(* Logix 5000 AddOnInstructionDefinition export SPEL_XYLimGet; software revision 30.01 *)

ADD_ON_INSTRUCTION SPEL_ExecCmd   (* revision 1.2 *)
// Executes a command in the robot controller.  Normally this is called by higher level AOIs.
VAR_INPUT
   Start : BOOL; {required}
   MaxTime : DINT := 3000; {required}
END_VAR
VAR_OUTPUT
   InCycle : BOOL; {access Read Only, visible}
   Done : BOOL; {access Read Only, visible}
   Error : BOOL; {access Read Only, visible}
END_VAR
VAR_IN_OUT
   ExtInputs : AB:ETHERNET_MODULE_INT_128Bytes:I:0; {required}
        .DATA[0].0   // ExtCmdGet
        .DATA[0].1   // ExtRespSet
        .DATA[0].2   // ExtCmdResult
        .DATA[0].3   // ExtError
   ExtOutputs : AB:ETHERNET_MODULE_INT_128Bytes:O:0; {required}
        .DATA[0].0   // ExtCmdSet
        .DATA[0].1   // ExtRespGet
        .DATA[0].2   // ExtCmdReset
END_VAR
VAR_INPUT
   Cmd : INT; {required}
   CmdParam1 : INT; {required}
   CmdParam2 : INT; {required}
   CmdParam3 : INT; {required}
   CmdParam4 : INT; {required}
   CmdParam5 : INT; {required}
   CmdParam6 : INT; {required}
   CmdParam7 : INT; {required}
END_VAR
VAR_OUTPUT
   CmdEcho : INT; {access Read Only, visible}
   Resp1 : INT; {access Read Only, visible}
   Resp2 : INT; {access Read Only, visible}
   Resp3 : INT; {access Read Only, visible}
   Resp4 : INT; {access Read Only, visible}
   Resp5 : INT; {access Read Only, visible}
   Resp6 : INT; {access Read Only, visible}
   Resp7 : INT; {access Read Only, visible}
   ErrCode1 : INT; {access Read Only, visible}
   ErrCode2 : INT; {access Read Only, visible}
END_VAR
VAR
   ExtReset : BOOL; {access None}
   ExtError : BOOL; {access None}
   ExtCmdSet : BOOL; {access None}   // Cmd Ready
   ExtCmdGet : BOOL; {access None}   // Cmd Received
   CmdXferDone : BOOL; {access None}
   ExtRespSet : BOOL; {access None}   // Resp Ready
   RespXferDone : BOOL; {access None}
   ExtCmdResult : BOOL; {access None}   // Normal or Error?
   TmrCmdDataRdy : TIMER := (PRE := 5); {access None}
   OneShotDoneOff : BOOL; {access None}
   OneShotStart : BOOL; {access None}
   StartInit : BOOL; {access None}
   OneShotStartError : BOOL; {access None}
   TmrCycle : TIMER := (PRE := 5000); {access None}
   OneshotTmrPreset : BOOL; {access None}
   TmrCmdSet : TIMER := (PRE := 20); {access None}
   OnShotCmdDataXfer : BOOL; {access None}
   OneShotRespDataXfer : BOOL; {access None}
   OneShotDataRdy : BOOL; {access None}
   OtherCmdInCycle : BOOL; {access None}
   s : BOOL; {access None}
   OneShotUnsetCmdIncycle : BOOL; {access None}
   OneShotSetCmdIncycle : BOOL; {access None}
   OneShotSetOtherCmdInCycleError : BOOL; {access None}
   OneShotSetBit : BOOL; {access None}
   MaxTimeError : BOOL; {access None}
END_VAR

ROUTINE Logic   (* ladder *)
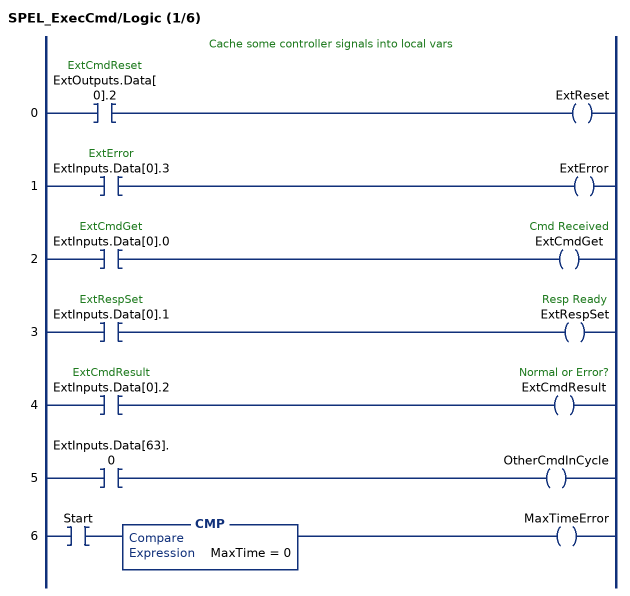
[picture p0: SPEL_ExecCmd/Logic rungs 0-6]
   // Cache some controller signals into local vars
   0: XIC(ExtOutputs.Data[0].2)OTE(ExtReset);
   1: XIC(ExtInputs.Data[0].3)OTE(ExtError);
   2: XIC(ExtInputs.Data[0].0)OTE(ExtCmdGet);
   3: XIC(ExtInputs.Data[0].1)OTE(ExtRespSet);
   4: XIC(ExtInputs.Data[0].2)OTE(ExtCmdResult);
   5: XIC(ExtInputs.Data[63].0)OTE(OtherCmdInCycle);
   6: XIC(Start)CMP(MaxTime = 0)OTE(MaxTimeError);
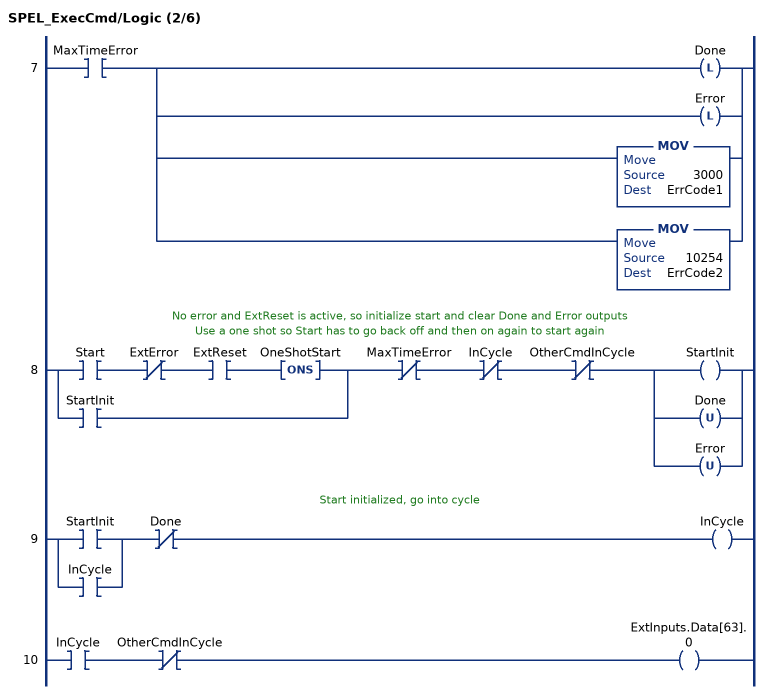
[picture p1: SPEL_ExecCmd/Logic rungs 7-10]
   7: XIC(MaxTimeError)[OTL(Done) ,OTL(Error) ,MOV(3000,ErrCode1) ,MOV(10254,ErrCode2) ];
   // No error and ExtReset is active, so initialize start and clear Done and Error outputs
   // Use a one shot so Start has to go back off and then on again to start again
   8: [XIC(Start) XIO(ExtError) XIC(ExtReset) ONS(OneShotStart) ,XIC(StartInit) ]XIO(MaxTimeError)XIO(InCycle)XIO(OtherCmdInCycle)[OTE(StartInit) ,OTU(Done) ,OTU(Error) ];
   // Start initialized, go into cycle
   9: [XIC(StartInit) ,XIC(InCycle) ]XIO(Done)OTE(InCycle);
   10: XIC(InCycle)XIO(OtherCmdInCycle)OTE(ExtInputs.Data[63].0);
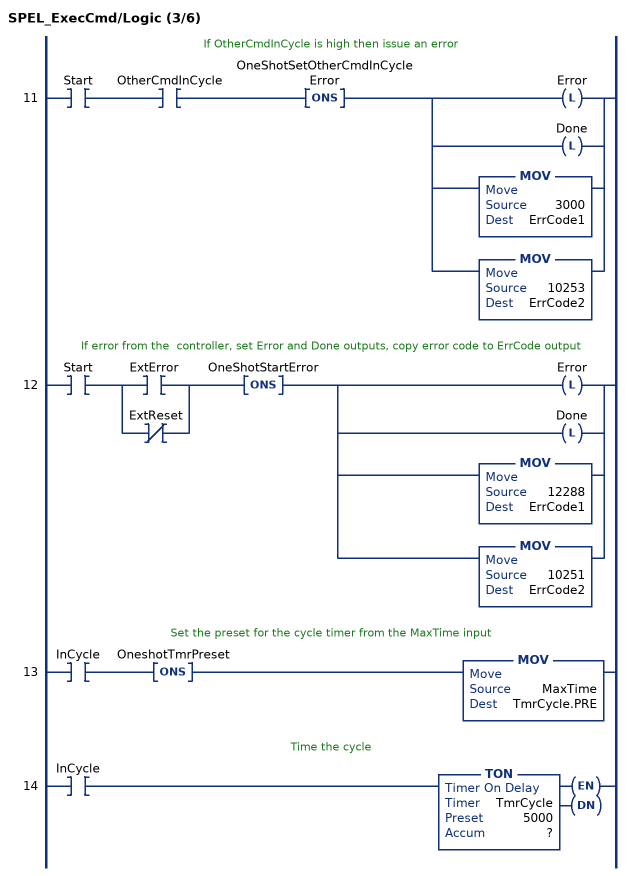
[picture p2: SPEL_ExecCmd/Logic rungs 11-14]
   // If OtherCmdInCycle is high then issue an error
   11: XIC(Start)XIC(OtherCmdInCycle)ONS(OneShotSetOtherCmdInCycleError)[OTL(Error) ,OTL(Done) ,MOV(3000,ErrCode1) ,MOV(10253,ErrCode2) ];
   // If error from the  controller, set Error and Done outputs, copy error code to ErrCode output
   12: XIC(Start)[XIC(ExtError) ,XIO(ExtReset) ]ONS(OneShotStartError)[OTL(Error) ,OTL(Done) ,MOV(12288,ErrCode1) ,MOV(10251,ErrCode2) ];
   // Set the preset for the cycle timer from the MaxTime input
   13: XIC(InCycle)ONS(OneshotTmrPreset)MOV(MaxTime,TmrCycle.PRE);
   // Time the cycle
   14: XIC(InCycle)TON(TmrCycle,?,?);
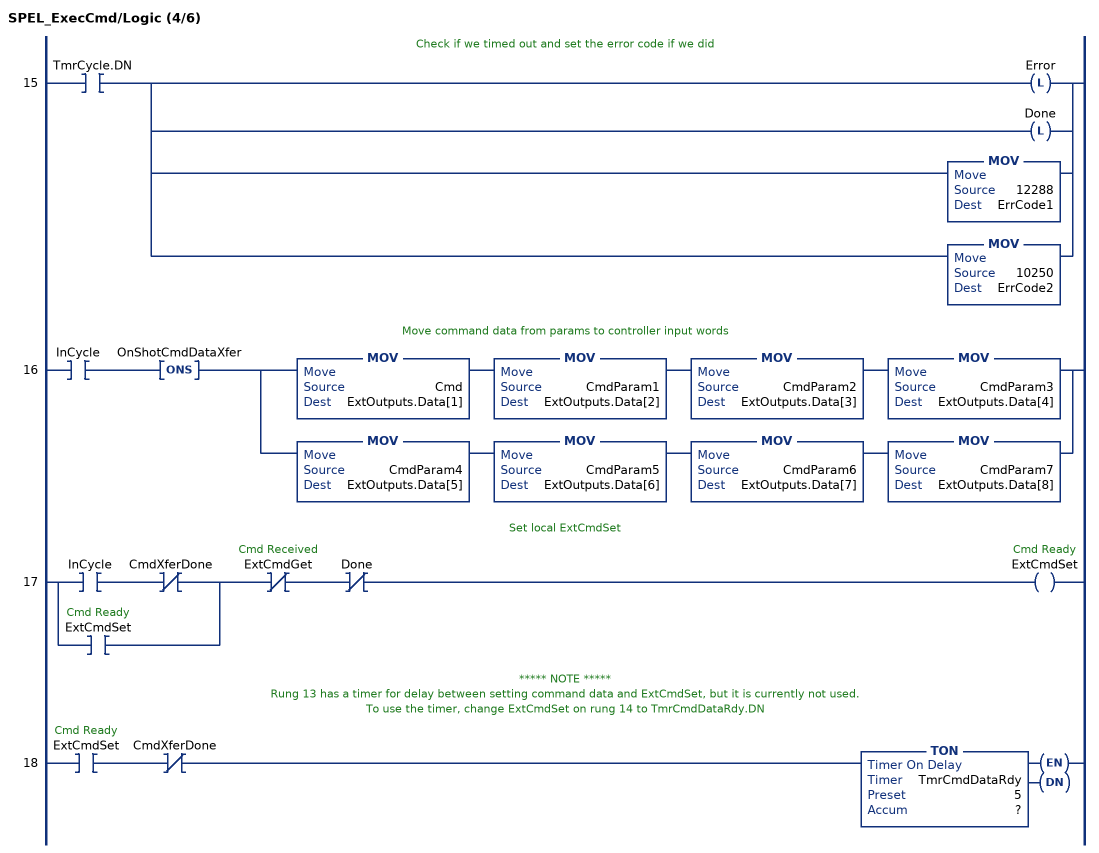
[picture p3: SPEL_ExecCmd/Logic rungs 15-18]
   // Check if we timed out and set the error code if we did
   15: XIC(TmrCycle.DN)[OTL(Error) ,OTL(Done) ,MOV(12288,ErrCode1) ,MOV(10250,ErrCode2) ];
   // Move command data from params to controller input words
   16: XIC(InCycle)ONS(OnShotCmdDataXfer)[MOV(Cmd,ExtOutputs.Data[1]) MOV(CmdParam1,ExtOutputs.Data[2]) MOV(CmdParam2,ExtOutputs.Data[3]) MOV(CmdParam3,ExtOutputs.Data[4]) ,MOV(CmdParam4,ExtOutputs.Data[5]) MOV(CmdParam5,ExtOutputs.Data[6]) MOV(CmdParam6,ExtOutputs.Data[7]) MOV(CmdParam7,ExtOutputs.Data[8]) ];
   // Set local ExtCmdSet
   17: [XIC(InCycle) XIO(CmdXferDone) ,XIC(ExtCmdSet) ]XIO(ExtCmdGet)XIO(Done)OTE(ExtCmdSet);
   // ***** NOTE *****
   // Rung 13 has a timer for delay between setting command data and ExtCmdSet, but it is currently not used.
   // To use the timer, change ExtCmdSet on rung 14 to TmrCmdDataRdy.DN
   18: XIC(ExtCmdSet)XIO(CmdXferDone)TON(TmrCmdDataRdy,?,?);
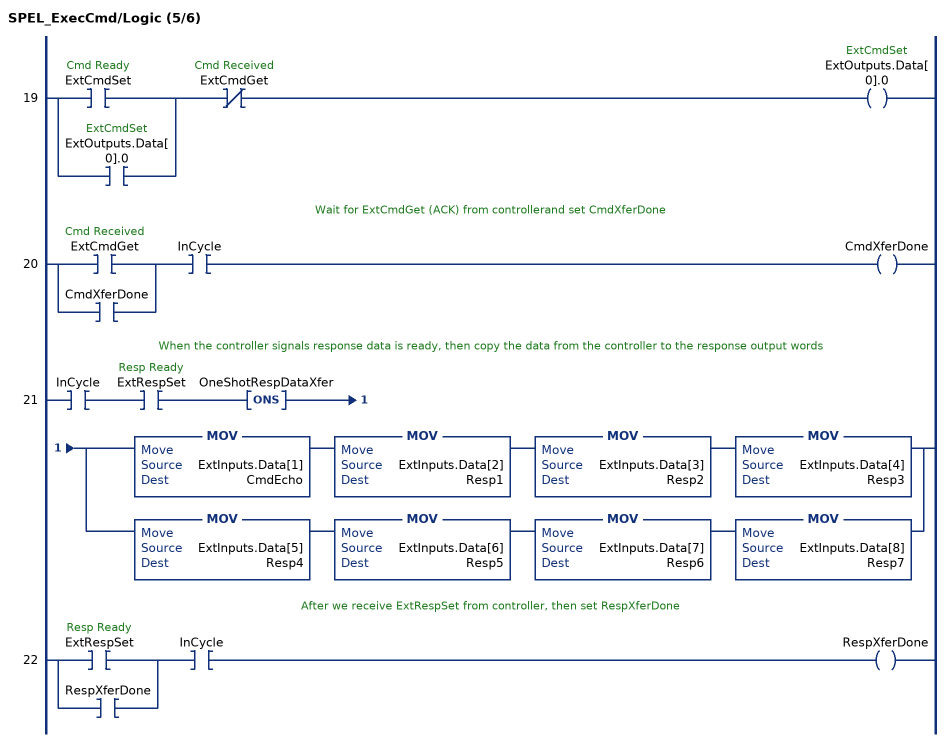
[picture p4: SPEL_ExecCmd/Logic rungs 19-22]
   19: [XIC(ExtCmdSet) ,XIC(ExtOutputs.Data[0].0) ]XIO(ExtCmdGet)OTE(ExtOutputs.Data[0].0);
   // Wait for ExtCmdGet (ACK) from controllerand set CmdXferDone
   20: [XIC(ExtCmdGet) ,XIC(CmdXferDone) ]XIC(InCycle)OTE(CmdXferDone);
   // When the controller signals response data is ready, then copy the data from the controller to the response output words
   21: XIC(InCycle)XIC(ExtRespSet)ONS(OneShotRespDataXfer)[MOV(ExtInputs.Data[1],CmdEcho) MOV(ExtInputs.Data[2],Resp1) MOV(ExtInputs.Data[3],Resp2) MOV(ExtInputs.Data[4],Resp3) ,MOV(ExtInputs.Data[5],Resp4) MOV(ExtInputs.Data[6],Resp5) MOV(ExtInputs.Data[7],Resp6) MOV(ExtInputs.Data[8],Resp7) ];
   // After we receive ExtRespSet from controller, then set RespXferDone
   22: [XIC(ExtRespSet) ,XIC(RespXferDone) ]XIC(InCycle)OTE(RespXferDone);
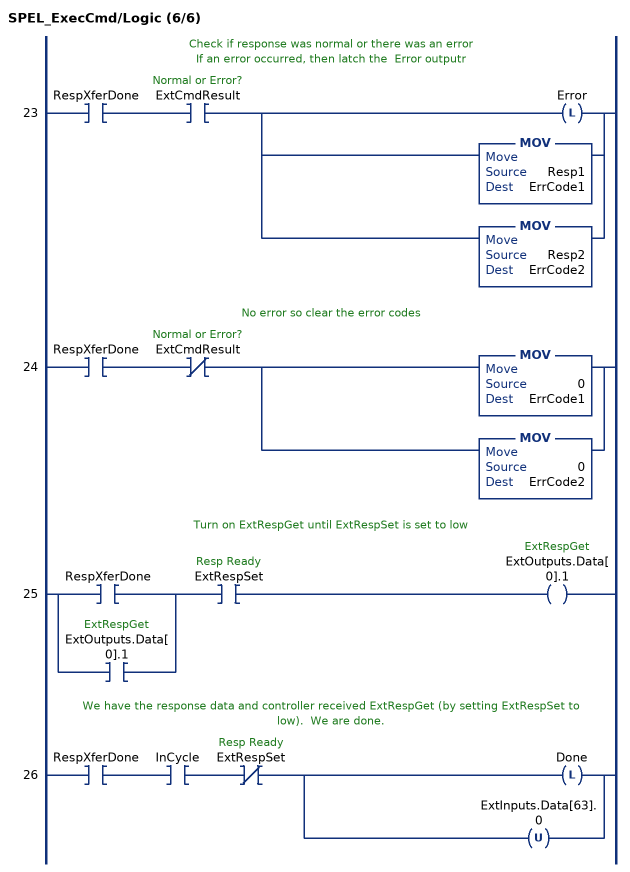
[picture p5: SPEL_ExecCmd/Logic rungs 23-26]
   // Check if response was normal or there was an error
   // If an error occurred, then latch the  Error outputr
   23: XIC(RespXferDone)XIC(ExtCmdResult)[OTL(Error) ,MOV(Resp1,ErrCode1) ,MOV(Resp2,ErrCode2) ];
   // No error so clear the error codes
   24: XIC(RespXferDone)XIO(ExtCmdResult)[MOV(0,ErrCode1) ,MOV(0,ErrCode2) ];
   // Turn on ExtRespGet until ExtRespSet is set to low
   25: [XIC(RespXferDone) ,XIC(ExtOutputs.Data[0].1) ]XIC(ExtRespSet)OTE(ExtOutputs.Data[0].1);
   // We have the response data and controller received ExtRespGet (by setting ExtRespSet to low).  We are done.
   26: XIC(RespXferDone)XIC(InCycle)XIO(ExtRespSet)[OTL(Done) ,OTU(ExtInputs.Data[63].0) ];
END_ROUTINE
END_ADD_ON_INSTRUCTION

ADD_ON_INSTRUCTION SPEL_XYLimGet   (* revision 1.2, vendor SEIKO EPSON CORP. *)
// Gets the setting value of the allowable motion
// area by specifying the lower and upper limit
// positions.
VAR_OUTPUT
   InCycle : BOOL; {access Read Only, visible}
   Done : BOOL; {access Read Only, visible}
   Error : BOOL; {access Read Only, visible}
END_VAR
VAR_INPUT
   Start : BOOL; {required}
END_VAR
VAR_OUTPUT
   XLower : REAL; {access Read Only, visible}
   XUpper : REAL; {access Read Only, visible}
   YLower : REAL; {access Read Only, visible}
   YUpper : REAL; {access Read Only, visible}
   ZLower : REAL; {access Read Only, visible}
   ZUpper : REAL; {access Read Only, visible}
END_VAR
VAR_IN_OUT
   ExtInputs : AB:ETHERNET_MODULE_INT_128Bytes:I:0; {required}
   ExtOutputs : AB:ETHERNET_MODULE_INT_128Bytes:O:0; {required}
END_VAR
VAR_OUTPUT
   ErrCode1 : INT; {access Read Only, visible}
   ErrCode2 : INT; {access Read Only, visible}
END_VAR
VAR
   ExecXYLimGetX : SPEL_ExecCmd := (MaxTime := 3000); {access None}
   lowerLimit_INTS : INT[2]; {access None}
   upperLimit_INTS : INT[2]; {access None}
   lowerLimitx1000 : DINT; {access None}
   upperLimitx1000 : DINT; {access None}
   StartInit : BOOL[32]; {access None}
   OneShotStart : BOOL[32]; {access None}
   ExecXYLimGetY : SPEL_ExecCmd := (MaxTime := 3000); {access None}
   ExecXYLimGetZ : SPEL_ExecCmd := (MaxTime := 3000); {access None}
   ExecTimeout : DINT; {access None}
END_VAR

ROUTINE Logic   (* ladder *)
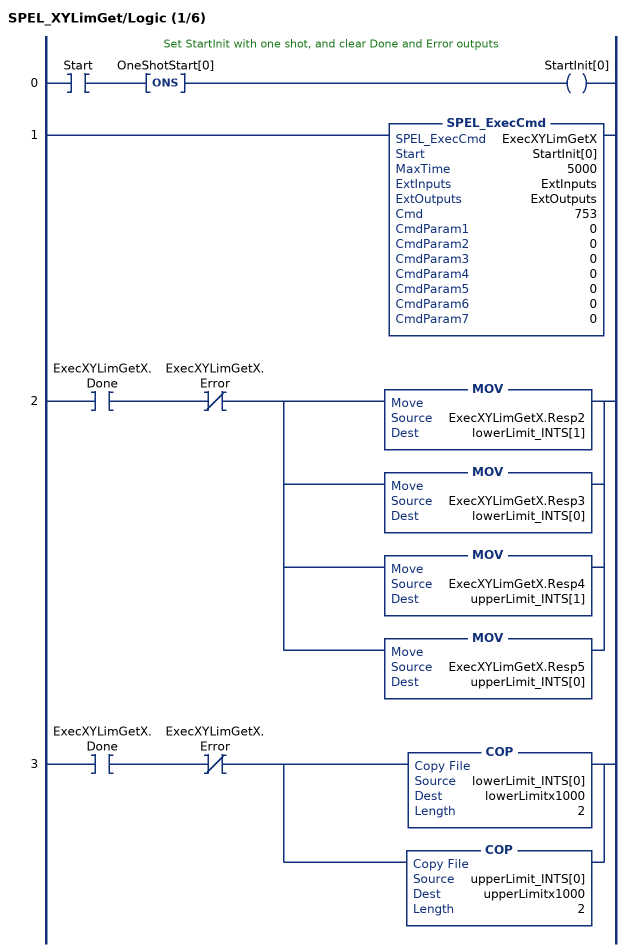
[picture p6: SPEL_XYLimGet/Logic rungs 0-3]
   // Set StartInit with one shot, and clear Done and Error outputs
   0: XIC(Start)ONS(OneShotStart[0])OTE(StartInit[0]);
   1: SPEL_ExecCmd(ExecXYLimGetX,StartInit[0],5000,ExtInputs,ExtOutputs,753,0,0,0,0,0,0,0);
   2: XIC(ExecXYLimGetX.Done)XIO(ExecXYLimGetX.Error)[MOV(ExecXYLimGetX.Resp2,lowerLimit_INTS[1]) ,MOV(ExecXYLimGetX.Resp3,lowerLimit_INTS[0]) ,MOV(ExecXYLimGetX.Resp4,upperLimit_INTS[1]) ,MOV(ExecXYLimGetX.Resp5,upperLimit_INTS[0]) ];
   3: XIC(ExecXYLimGetX.Done)XIO(ExecXYLimGetX.Error)[COP(lowerLimit_INTS[0],lowerLimitx1000,2) ,COP(upperLimit_INTS[0],upperLimitx1000,2) ];
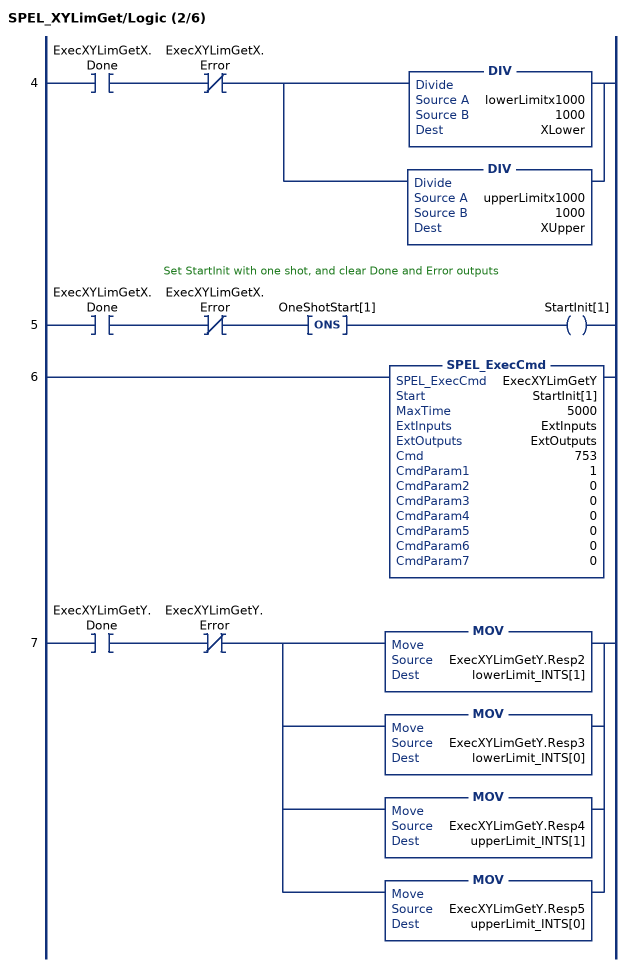
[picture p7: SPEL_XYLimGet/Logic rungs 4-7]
   4: XIC(ExecXYLimGetX.Done)XIO(ExecXYLimGetX.Error)[DIV(lowerLimitx1000,1000,XLower) ,DIV(upperLimitx1000,1000,XUpper) ];
   // Set StartInit with one shot, and clear Done and Error outputs
   5: XIC(ExecXYLimGetX.Done)XIO(ExecXYLimGetX.Error)ONS(OneShotStart[1])OTE(StartInit[1]);
   6: SPEL_ExecCmd(ExecXYLimGetY,StartInit[1],5000,ExtInputs,ExtOutputs,753,1,0,0,0,0,0,0);
   7: XIC(ExecXYLimGetY.Done)XIO(ExecXYLimGetY.Error)[MOV(ExecXYLimGetY.Resp2,lowerLimit_INTS[1]) ,MOV(ExecXYLimGetY.Resp3,lowerLimit_INTS[0]) ,MOV(ExecXYLimGetY.Resp4,upperLimit_INTS[1]) ,MOV(ExecXYLimGetY.Resp5,upperLimit_INTS[0]) ];
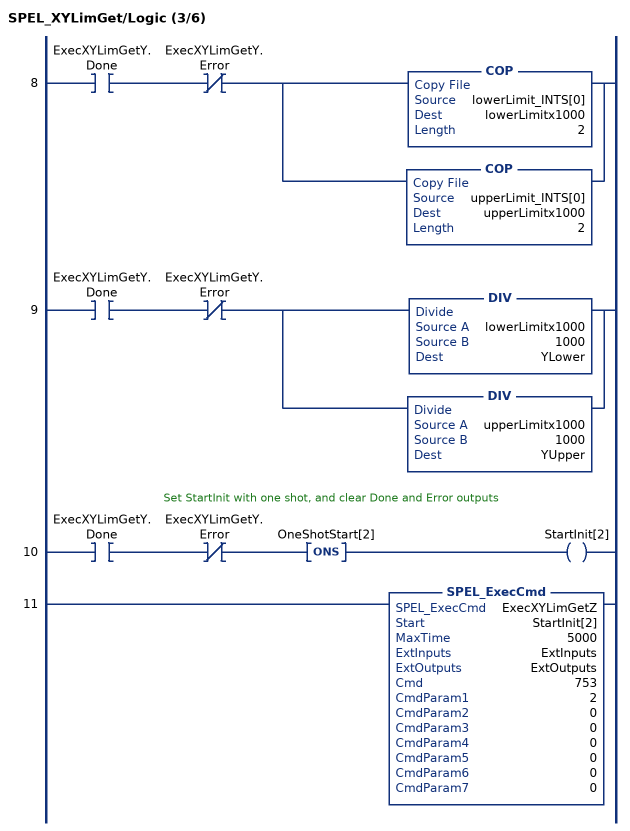
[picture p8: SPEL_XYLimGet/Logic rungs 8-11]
   8: XIC(ExecXYLimGetY.Done)XIO(ExecXYLimGetY.Error)[COP(lowerLimit_INTS[0],lowerLimitx1000,2) ,COP(upperLimit_INTS[0],upperLimitx1000,2) ];
   9: XIC(ExecXYLimGetY.Done)XIO(ExecXYLimGetY.Error)[DIV(lowerLimitx1000,1000,YLower) ,DIV(upperLimitx1000,1000,YUpper) ];
   // Set StartInit with one shot, and clear Done and Error outputs
   10: XIC(ExecXYLimGetY.Done)XIO(ExecXYLimGetY.Error)ONS(OneShotStart[2])OTE(StartInit[2]);
   11: SPEL_ExecCmd(ExecXYLimGetZ,StartInit[2],5000,ExtInputs,ExtOutputs,753,2,0,0,0,0,0,0);
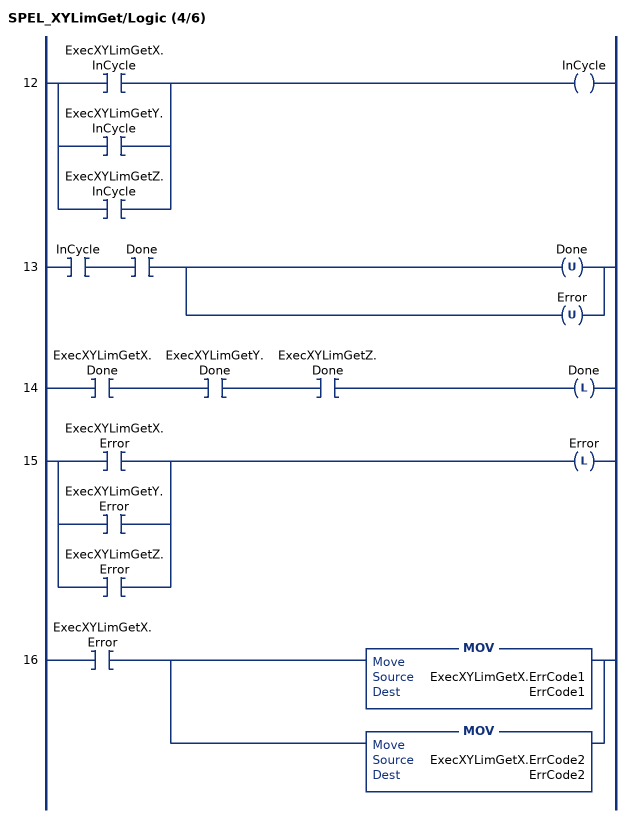
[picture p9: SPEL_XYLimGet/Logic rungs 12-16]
   12: [XIC(ExecXYLimGetX.InCycle) ,XIC(ExecXYLimGetY.InCycle) ,XIC(ExecXYLimGetZ.InCycle) ]OTE(InCycle);
   13: XIC(InCycle)XIC(Done)[OTU(Done) ,OTU(Error) ];
   14: XIC(ExecXYLimGetX.Done)XIC(ExecXYLimGetY.Done)XIC(ExecXYLimGetZ.Done)OTL(Done);
   15: [XIC(ExecXYLimGetX.Error) ,XIC(ExecXYLimGetY.Error) ,XIC(ExecXYLimGetZ.Error) ]OTL(Error);
   16: XIC(ExecXYLimGetX.Error)[MOV(ExecXYLimGetX.ErrCode1,ErrCode1) ,MOV(ExecXYLimGetX.ErrCode2,ErrCode2) ];
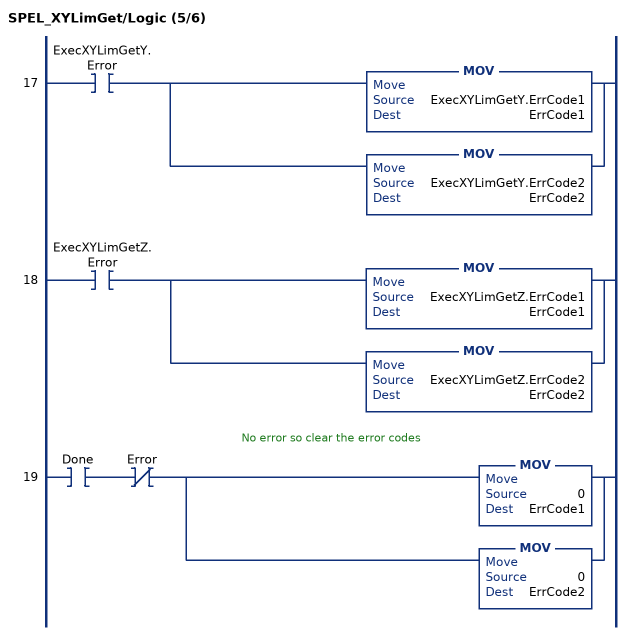
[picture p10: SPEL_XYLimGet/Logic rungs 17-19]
   17: XIC(ExecXYLimGetY.Error)[MOV(ExecXYLimGetY.ErrCode1,ErrCode1) ,MOV(ExecXYLimGetY.ErrCode2,ErrCode2) ];
   18: XIC(ExecXYLimGetZ.Error)[MOV(ExecXYLimGetZ.ErrCode1,ErrCode1) ,MOV(ExecXYLimGetZ.ErrCode2,ErrCode2) ];
   // No error so clear the error codes
   19: XIC(Done)XIO(Error)[MOV(0,ErrCode1) ,MOV(0,ErrCode2) ];
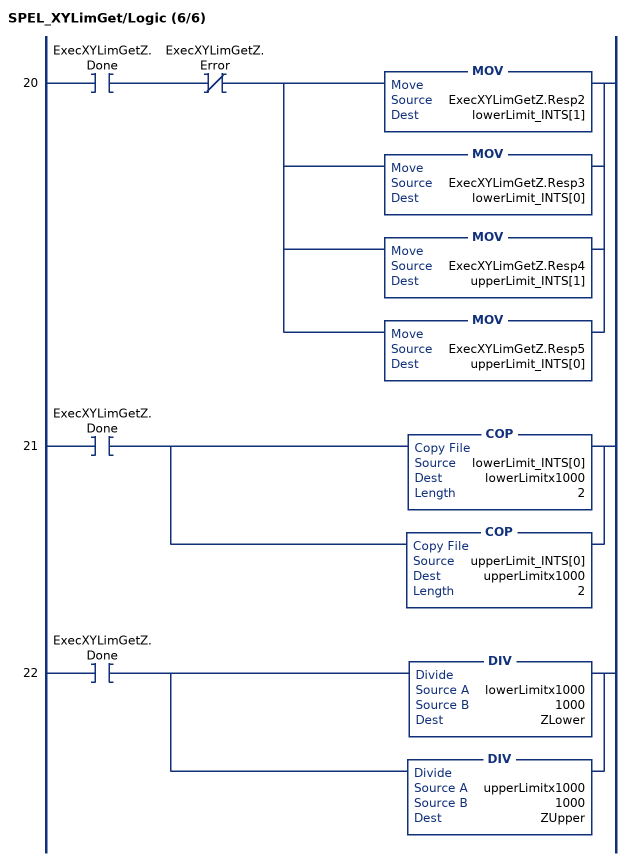
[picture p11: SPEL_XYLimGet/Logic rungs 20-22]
   20: XIC(ExecXYLimGetZ.Done)XIO(ExecXYLimGetZ.Error)[MOV(ExecXYLimGetZ.Resp2,lowerLimit_INTS[1]) ,MOV(ExecXYLimGetZ.Resp3,lowerLimit_INTS[0]) ,MOV(ExecXYLimGetZ.Resp4,upperLimit_INTS[1]) ,MOV(ExecXYLimGetZ.Resp5,upperLimit_INTS[0]) ];
   21: XIC(ExecXYLimGetZ.Done)[COP(lowerLimit_INTS[0],lowerLimitx1000,2) ,COP(upperLimit_INTS[0],upperLimitx1000,2) ];
   22: XIC(ExecXYLimGetZ.Done)[DIV(lowerLimitx1000,1000,ZLower) ,DIV(upperLimitx1000,1000,ZUpper) ];
END_ROUTINE
END_ADD_ON_INSTRUCTION
